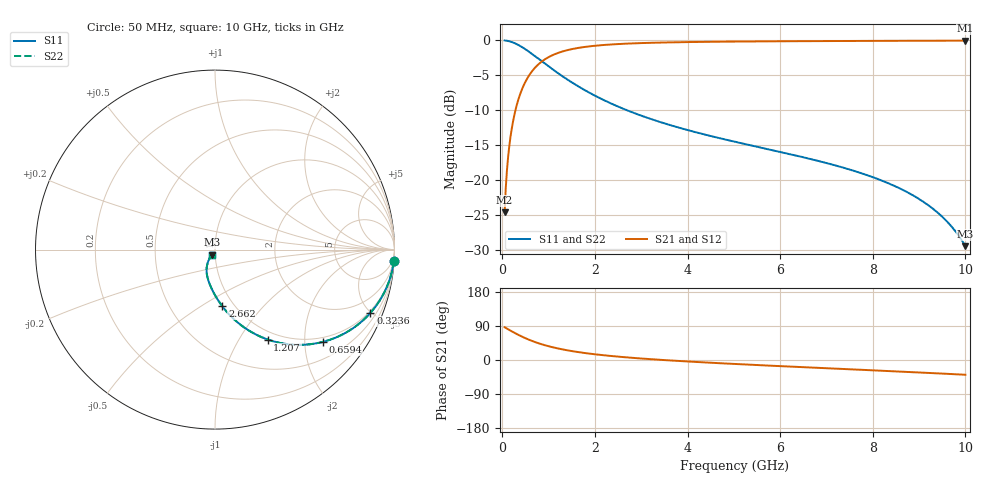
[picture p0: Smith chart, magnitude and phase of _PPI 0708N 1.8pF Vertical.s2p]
! S-Parameter data specifications (vertical orientation):
! Substrate: 40-mil Rogers 3003C, Substrate thickness, H=1.016mm, Dielectric constant, Er=3, Conductor thickness, T_mtl=0.043mm, Loss Tangent, Tand=0.003
! PCB Mounting Pad Footprint: Pad width, PadW=2.54mm , Pad length, PadL=0.51mm , Pad gap, PadG (edge-to-edge)=0.71mm , Reference planes=1.73mm apart
! Created Tue Jan 16 08:43:53 2018
# GHz S MA R 50
! 2 Port Network Data from SP1.SP block
! freq  magS11  angS11  magS21  angS21  magS12  angS12  magS22  angS22
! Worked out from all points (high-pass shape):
!   801 points, 50 MHz to 10 GHz, reference 50 ohm
!   highest |S21| = -0.04 dB at 10 GHz (marker M1); lowest = -24.6 dB at 50 MHz (marker M2)
!   |S21| within 3 dB of the highest: 851.2 MHz to end of sweep
!   lowest |S11| = -29.5 dB at 10 GHz (marker M3), VSWR 1.07, Z = 48.2 - j2.74 ohm
!   |S11| at or under -10 dB: 2.687 GHz to end of sweep
!   |S22| runs from -29.5 to 0.0 dB; largest |S21 - S12| = 0
!   S11 on the Smith chart (normalised r, x): 50 MHz: 1, -32; 323.6 MHz: 0.88, -4.95; 659.4 MHz: 0.88, -2.43; 1.207 GHz: 0.88, -1.34; 2.662 GHz: 0.88, -0.62; 10 GHz: 0.96, -0.05
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0.05  0.9983 -3.6  0.0586 86.4  0.0586 86.4  0.9983 -3.6
0.074875  0.9962 -5.3  0.08756 84.7  0.08756 84.7  0.9962 -5.3
0.124625  0.9894 -8.9  0.1447 81.1  0.1447 81.1  0.9894 -8.9
0.174375  0.9797 -12.3  0.2005 77.7  0.2005 77.7  0.9797 -12.3
0.2365625  0.9635 -16.5  0.2675 73.5  0.2675 73.5  0.9635 -16.5
0.323625  0.9348 -22.2  0.3549 67.8  0.3549 67.8  0.9348 -22.2
0.472875  0.8745 -31.0  0.4846 59.0  0.4846 59.0  0.8745 -31.0
0.6594375  0.7916 -40.5  0.6106 49.5  0.6106 49.5  0.7916 -40.5
0.9330625  0.6765 -51.4  0.7358 38.5  0.7358 38.5  0.6765 -51.4
1.206687  0.5808 -59.6  0.8133 30.3  0.8133 30.3  0.5808 -59.6
1.443  0.5141 -65.2  0.8568 24.7  0.8568 24.7  0.5141 -65.2
1.716625  0.4523 -70.4  0.8909 19.5  0.8909 19.5  0.4523 -70.4
2.1395  0.3806 -76.7  0.9236 13.2  0.9236 13.2  0.3806 -76.7
2.661875  0.3186 -82.6  0.9466 7.2  0.9466 7.2  0.3186 -82.6
3.370812  0.2623 -88.9  0.9635 0.8  0.9635 0.8  0.2623 -88.9
5.025  0.1876 -100.0  0.9803 -10.5  0.9803 -10.5  0.1876 -100.0
6.691625  0.1403 -109.1  0.9876 -20.0  0.9876 -20.0  0.1403 -109.1
8.345812  0.09439 -117.4  0.9923 -29.2  0.9923 -29.2  0.09439 -117.4
8.880625  0.07711 -119.9  0.9935 -32.2  0.9935 -32.2  0.07711 -119.9
9.328375  0.06108 -121.6  0.9943 -34.8  0.9943 -34.8  0.06108 -121.6
9.676625  0.04737 -122.5  0.9948 -36.9  0.9948 -36.9  0.04737 -122.5
10  0.03353 -122.2  0.9951 -38.9  0.9951 -38.9  0.03353 -122.2
